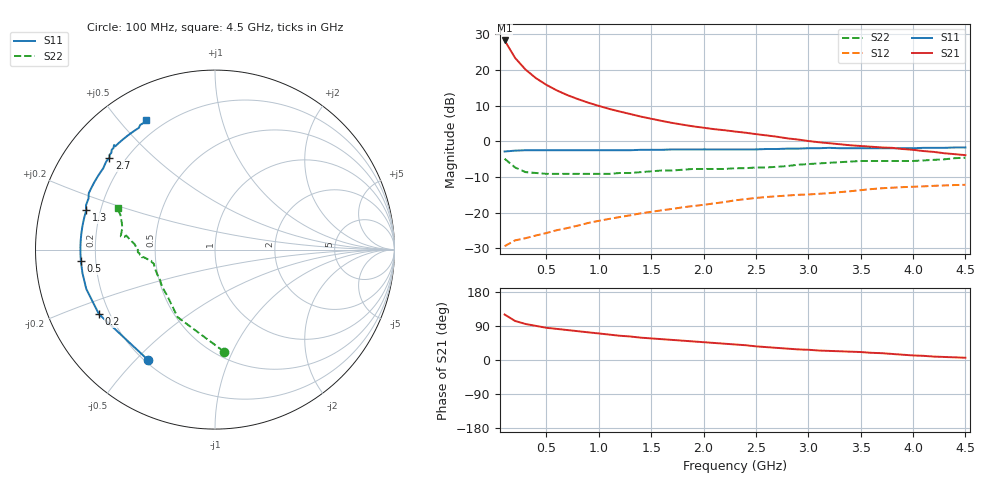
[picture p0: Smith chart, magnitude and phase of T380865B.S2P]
!AT-38086
!S-PARAMETERS at Vce=4.8V  Ic=50mA.  LAST UPDATED 08-05-96
# ghz s ma r 50
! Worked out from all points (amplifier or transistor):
!   45 points, 100 MHz to 4.5 GHz, reference 50 ohm
!   highest |S21| = 28.2 dB at 100 MHz (marker M1)
!   |S21| within 3 dB of that: start of sweep to 161.5 MHz
!   unconditionally stable (mu >= 1): 888 MHz to end of sweep
!   at 800 MHz: K = 0.97, MSG = 17.7 dB, |S12| = -23.6 dB
!   at 2.3 GHz: K = 1.11, MAG = 7.6 dB, |S12| = -16.5 dB
!   at 4.5 GHz: K = 1.08, MAG = 2.4 dB, |S12| = -12.2 dB
!   S11 on the Smith chart (normalised r, x): 100 MHz: 0.21, -0.55; 200 MHz: 0.16, -0.25; 500 MHz: 0.14, -0.04; 1.3 GHz: 0.15, +0.15; 2.7 GHz: 0.14, +0.37; 4.5 GHz: 0.13, +0.59
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0.1  0.72 -121.0  25.84 120.0  0.034 41.0  0.57 -85.0
0.2  0.74 -151.0  14.73 103.0  0.041 34.0  0.43 -119.0
0.3  0.75 -163.0  10.09 95.0  0.044 36.0  0.37 -136.0
0.4  0.75 -170.0  7.65 90.0  0.048 39.0  0.36 -145.0
0.5  0.75 -175.0  6.16 85.0  0.052 42.0  0.35 -151.0
0.6  0.75 -178.0  5.15 82.0  0.057 45.0  0.35 -156.0
0.7  0.75 179.0  4.43 79.0  0.061 48.0  0.35 -159.0
0.8  0.75 176.0  3.9 76.0  0.066 50.0  0.35 -161.0
0.9  0.75 173.0  3.47 73.0  0.072 51.0  0.35 -164.0
1  0.75 170.0  3.13 70.0  0.077 53.0  0.35 -165.0
1.1  0.75 168.0  2.84 67.0  0.082 54.0  0.35 -167.0
1.2  0.75 166.0  2.61 64.0  0.087 55.0  0.36 -169.0
1.3  0.75 163.0  2.41 62.0  0.092 55.0  0.36 -170.0
1.4  0.76 161.0  2.22 59.0  0.098 56.0  0.37 -171.0
1.6  0.76 158.0  1.93 55.0  0.108 57.0  0.39 -173.0
1.9  0.77 154.0  1.62 49.0  0.124 57.0  0.41 -174.0
2.3  0.77 148.0  1.37 41.0  0.149 57.0  0.42 -176.0
2.7  0.78 139.0  1.16 32.0  0.17 54.0  0.44 178.0
3.1  0.8 135.0  0.97 25.0  0.184 52.0  0.49 172.0
3.5  0.8 132.0  0.86 21.0  0.207 51.0  0.53 172.0
3.8  0.8 126.0  0.81 16.0  0.224 48.0  0.53 170.0
4.5  0.82 118.0  0.64 6.0  0.246 41.0  0.59 157.0
